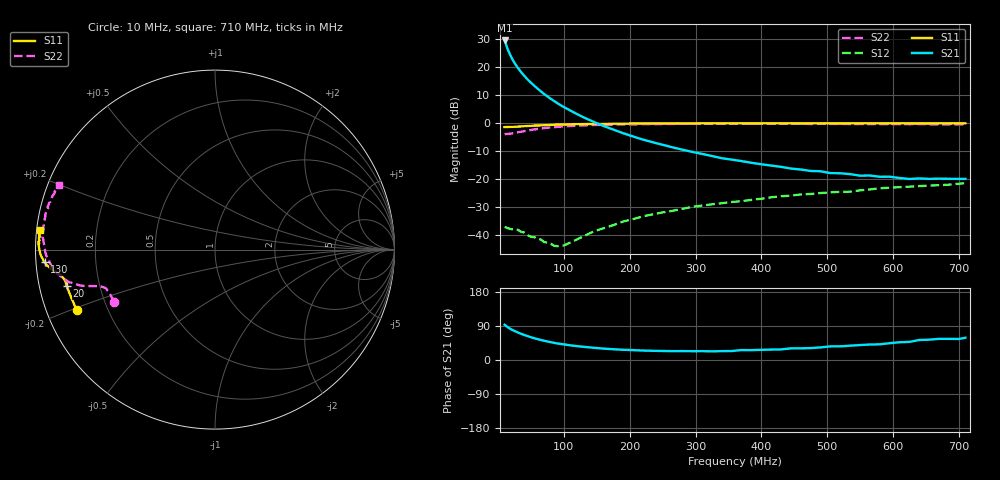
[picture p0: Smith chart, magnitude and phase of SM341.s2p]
!  POLYFET RF DEVICES
!  SM341
!  S PARAMETERS
!  VDS=50V, IDQ=600mA
# MHZ S MA R 50
! Freq=Mhz Mag[s11] Ang[s11] Mag[s21] Ang[s21] Mag[s12] Ang[s12] Mag[s22] Ang[s22]
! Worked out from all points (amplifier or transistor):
!   60 points, 10 MHz to 710 MHz, reference 50 ohm
!   highest |S21| = 29.3 dB at 10 MHz (marker M1)
!   |S21| within 3 dB of that: start of sweep to 14.56 MHz
!   unconditionally stable (mu >= 1): 532.2 MHz to end of sweep
!   at 60 MHz: K = 0.49, MSG = 26.8 dB, |S12| = -41.3 dB
!   at 280 MHz: K = 0.57, MSG = 10.5 dB, |S12| = -30.6 dB
!   at 710 MHz: K = 1.16, MAG = -1.7 dB, |S12| = -21.5 dB
!   S11 on the Smith chart (normalised r, x): 10 MHz: 0.09, -0.21; 20 MHz: 0.08, -0.12; 130 MHz: 0.02, -0.04; 710 MHz: 0.01, +0.06
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10  0.8418 -156.3  29.33 93.0  0.01411 7.0  0.6318 -152.7
15  0.8462 -162.9  20.08 86.1  0.01338 4.5  0.637 -158.4
20  0.8506 -166.3  14.86 81.0  0.01282 0.1  0.6473 -160.8
25  0.8526 -168.1  11.74 76.5  0.01294 0.3  0.6653 -161.9
30  0.8581 -169.2  9.581 72.8  0.01254 -1.2  0.6795 -162.5
35  0.867 -170.1  8.021 69.2  0.01155 -4.5  0.696 -163.0
40  0.8735 -170.7  6.865 66.0  0.01118 -3.9  0.7139 -163.4
45  0.8816 -171.1  5.912 62.9  0.01006 -3.9  0.7296 -163.8
50  0.886 -171.6  5.203 60.0  0.00936 -1.4  0.7482 -164.2
55  0.8942 -171.8  4.585 57.6  0.00927 -3.4  0.7652 -164.7
60  0.8995 -172.2  4.088 55.1  0.00863 1.1  0.7807 -165.2
70  0.9095 -172.8  3.27 50.8  0.0076 9.7  0.8072 -166.3
85  0.9263 -173.7  2.457 45.3  0.00651 27.2  0.8398 -167.9
100  0.937 -174.4  1.915 41.2  0.00659 39.8  0.8643 -169.7
115  0.9472 -175.2  1.54 37.5  0.00791 61.7  0.8892 -171.3
130  0.9523 -175.7  1.255 34.8  0.00963 71.6  0.9034 -172.8
175  0.9661 -177.4  0.7613 28.4  0.01515 80.8  0.9324 -176.9
250  0.9758 -179.5  0.4078 23.8  0.02554 88.2  0.9558 177.5
370  0.9842 178.1  0.209 26.3  0.04051 88.6  0.9645 170.9
490  0.9841 176.4  0.1378 33.3  0.05653 87.9  0.9626 165.8
595  0.9809 174.9  0.1103 44.4  0.07044 87.6  0.9524 161.6
710  0.9822 173.6  0.1009 58.8  0.08459 89.1  0.9422 157.5
